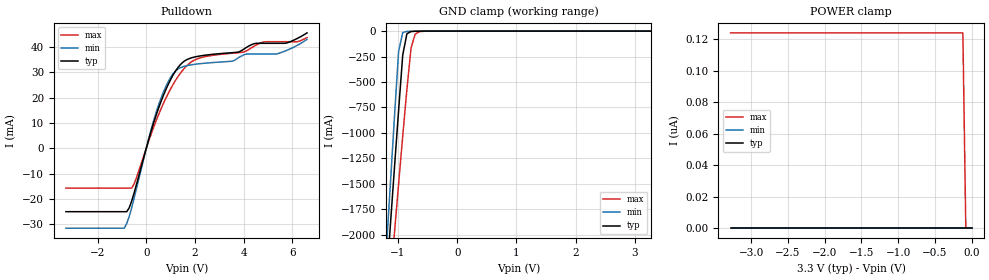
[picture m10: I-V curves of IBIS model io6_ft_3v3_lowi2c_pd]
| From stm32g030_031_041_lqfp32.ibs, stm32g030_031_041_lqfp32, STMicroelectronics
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[Model]  io6_ft_3v3_lowi2c_pd
Model_type I/O_open_drain
Polarity   Non-Inverting
Enable   Active-Low
Vinl =   0.990000V
Vinh =   2.310000V
Vmeas =  1.650000V
Cref =   50.000000pF
Rref =   500
Vref =   3.0V
C_comp   1.290400pF   1.272500pF   1.305600pF
[Temperature Range]   25.000000   -40.000000   0.125000k
[Pullup Reference]   3.300000V   3.000000V   3.600000V
[Pulldown Reference]   0.0V   0.0V   0.0V
[POWER Clamp Reference]   3.300000V   3.000000V   3.600000V
[GND Clamp Reference]   0.0V   0.0V   0.0V
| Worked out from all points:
|   slope of the pulldown table from 0 to 0.495 V, typ, clamps not added: 31.8 ohm
|   GND clamp passes 1 mA (typ) near -0.65 V on its own axis
[Pulldown]
|Voltage   I(typ)   I(min)   I(max)
-3.3V     -25.03mA   -31.54mA   -15.7mA
-900mV    -25.03mA   -31.54mA   -15.7mA
-700mV    -23.48mA   -26.95mA   -15.7mA
-500mV    -17.69mA   -19.75mA   -14.07mA
100mV     3.479mA    3.853mA    2.862mA
500mV     15.71mA    16.96mA    13.17mA
900mV     25.22mA    26.33mA    21.66mA
1.3V      31.91mA    31.32mA    28.29mA
2.2V      36.48mA    33.43mA    35.69mA
4.1V      39.78mA    37.21mA    38.43mA
5.4V      41.49mA    37.39mA    42.11mA
6.6V      45.6mA     43.05mA    43.74mA
[GND_clamp]
|Voltage   I(typ)   I(min)   I(max)
-3.3V     -9.61A     -9.635A    -9.699A
-1.2V     -2.493A    -2.184A    -2.958A
-1.13V    -1.917A    -1.512A    -2.469A
-1.06V    -1.345A    -845.6mA   -1.983A
-990mV    -779.8mA   -200.2mA   -1.503A
-920mV    -235.6mA   -14.2mA    -1.03A
-850mV    -26.08mA   -3.351mA   -574.2mA
-780mV    -4.512mA   -1.821mA   -166.4mA
-710mV    -1.735mA   -881.8uA   -29.46mA
-640mV    -819.4uA   -295.6uA   -6.294mA
3.28V     86.85uA    64.2uA     109.1uA
[POWER_clamp]
|Voltage   I(typ)   I(min)   I(max)
-3.28V    0A         0A         124nA
-120mV    0A         0A         124nA
-80mV     0A         0A         0A
0V        0A         0A         0A
[Ramp]
| variable   typ   min   max
dV/dt_r  1.07424/45.63765n   0.96276/40.30836n   1.028/56.91530n
dV/dt_f  1.03170/40.74641n   0.95310/40.32798n   1.02444/43.53390n
R_load = 50.000000
